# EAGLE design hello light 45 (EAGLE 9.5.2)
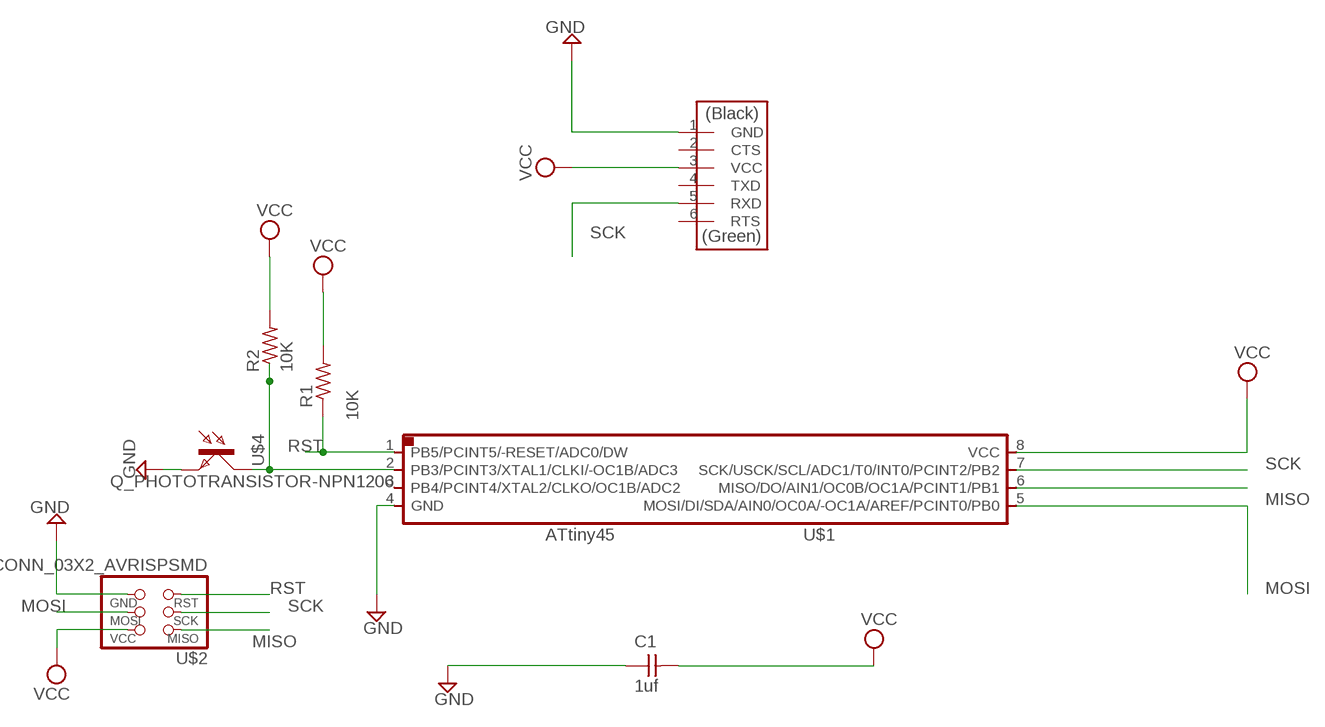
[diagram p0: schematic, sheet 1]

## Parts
C1  1uf  CAP_UNPOLARIZED  [C1206]
R1  10K  R1206FAB  [R1206FAB]
R2  10K  R1206FAB  [R1206FAB]
U$1  UC_ATTINY45SI  [SOIC8]
U$2  CONN_03X2_AVRISPSMD  [2X03SMD]
U$3  CONN_06_FTDI-SMD-HEADER  [1X06SMD]
U$4  Q_PHOTOTRANSISTOR-NPN1206  [OP1206]

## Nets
GND: C1.1 U$1.4(GND) U$2.6(GND) U$3.1(GND) U$4.EMITTER(E)
MISO: U$1.6(MISO/DO/AIN1/OC0B/OC1A/PCINT1/PB1) U$2.1(MISO)
MOSI: U$1.5(MOSI/DI/SDA/AIN0/OC0A/-OC1A/AREF/PCINT0/PB0) U$2.4(MOSI)
N$2: R2.1 U$1.2(PB3/PCINT3/XTAL1/CLKI/-OC1B/ADC3) U$4.COLLECTOR(C)
RST: R1.1 U$1.1(PB5/PCINT5/-RESET/ADC0/DW) U$2.5(RST)
SCK: U$1.7(SCK/USCK/SCL/ADC1/T0/INT0/PCINT2/PB2) U$2.3(SCK) U$3.5(RXD)
VCC: C1.2 R1.2 R2.2 U$1.8(VCC) U$2.2(VCC) U$3.3(VCC)
Unconnected: U$1.3(PB4/PCINT4/XTAL2/CLKO/OC1B/ADC2) U$3.2(CTS) U$3.4(TXD) U$3.6(RTS)

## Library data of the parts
C1 = fab:CAP_UNPOLARIZED
R1 R2 = fab:R: Resistor (US Symbol)
U$1 = fab:UC_ATTINY45
U$2 = fab:CONN_03X2_AVRISP
U$3 = fab:CONN_06_FTDI-SMD-HEADER
U$4 = fab:Q_PHOTOTRANSISTOR-NPN

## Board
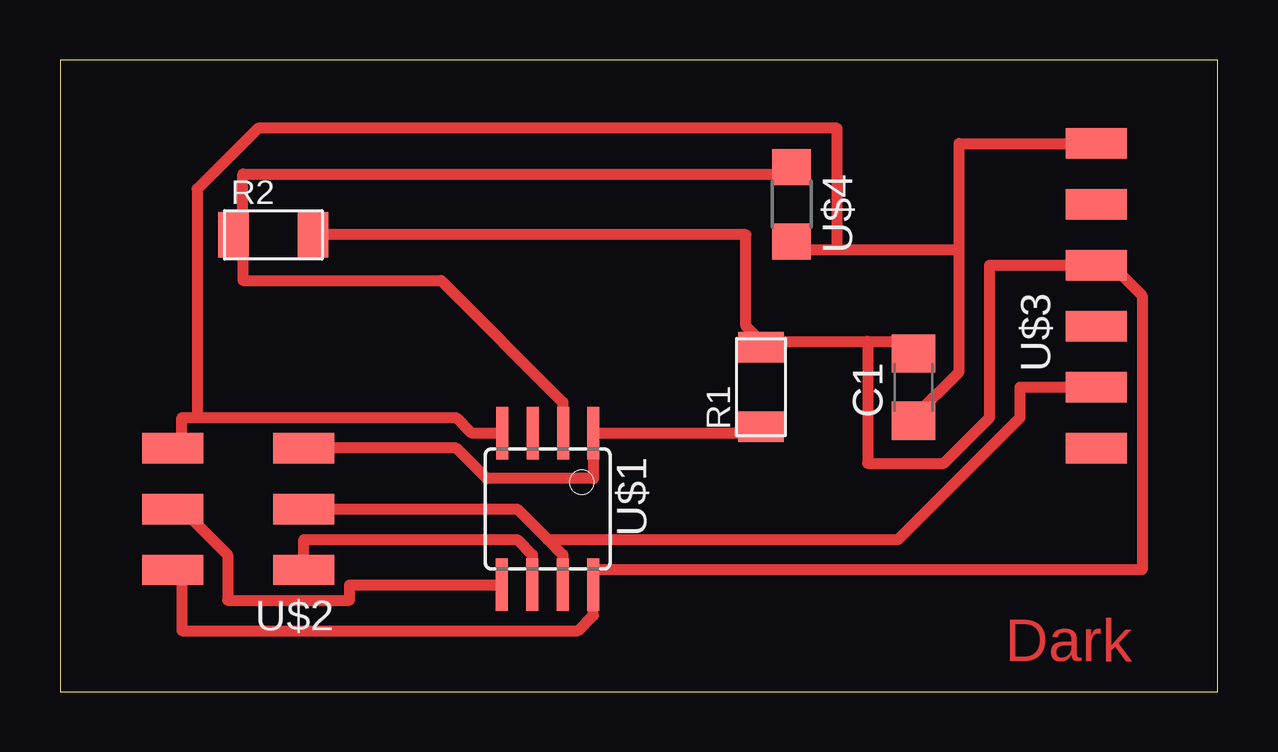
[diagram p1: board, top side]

Size 48.24 x 26.34 mm. Coordinates in mm from the lower left corner, seen from the top.
Outline: 0,0 48.24,0 48.24,26.34 0,26.34 0,0
Copper layers (1*16): Top 0.035mm / dielectric 1.5mm / Bottom 0.035mm
Design rules "fab-1": minimum track width 0.45mm, minimum drill 32mil, track to track 16mil, track to pad 16mil, pad to pad 16mil, via to via 16mil, smd to smd 6mil, copper to edge 16mil, drill to drill 16mil, minimum pad ring 10mil, minimum via ring 8mil, stop-mask expansion 4mil, vias tented up to drill 0mil, thermal gap 16mil

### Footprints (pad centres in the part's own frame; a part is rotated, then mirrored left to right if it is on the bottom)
C1206 = smd 1.6 x 1.8: 1 -1.4,0; 2 1.4,0
R1206FAB = smd 1.27 x 1.905: 1 -1.651,0; 2 1.651,0
SOIC8 = smd 0.5 x 2.2: 1 -1.905,-3.154; 2 -0.645,-3.154; 3 0.625,-3.154; 4 1.895,-3.154; 5 1.905,3.154; 6 0.635,3.154; 7 -0.635,3.154; 8 -1.905,3.154
2X03SMD = smd 2.54 x 1.27: 1 -2.54,2.54; 2 2.92,2.54; 3 -2.54,0; 4 2.92,0; 5 -2.54,-2.54; 6 2.92,-2.54
1X06SMD = smd 2.54 x 1.27: 1 0,6.35; 2 0,3.81; 3 0,1.27; 4 0,-1.27; 5 0,-3.81; 6 0,-6.35
OP1206 = smd 1.5 x 1.6: COLLECTOR -1.55,0; EMITTER 1.55,0

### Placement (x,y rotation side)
C1  35.56,12.7 90 top
R1  29.21,12.7 90 top
R2  8.89,19.05 0 top
U$1  20.32,7.62 180 top
U$2  7.62,7.62 180 top
U$3  43.18,16.51 0 top
U$4  30.48,20.32 270 top

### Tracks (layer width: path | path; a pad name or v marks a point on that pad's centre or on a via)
GND
  Top 0.45: 5.71,11.43 5.08,11.43 5.08,10.16 U$2.6 | 5.71,11.43 16.51,11.43 17.14,10.79 18.41,10.79 U$1.4 | 37.47,18.41 32.38,18.41 | 32.38,18.41 30.48,18.41 U$4.EMITTER | 37.47,18.41 37.47,13.34 35.56,11.43 C1.1 | U$3.1 37.47,22.86 37.47,18.41 | 5.71,11.43 5.71,20.95 8.25,23.49 32.38,23.49 32.38,18.41
MISO
  Top 0.45: U$1.6 19.68,5.71 19.05,6.35 10.16,6.35 U$2.1
MOSI
  Top 0.45: U$1.5 18.41,4.45 12.06,4.45 12.06,3.81 6.98,3.81 6.98,5.71 5.08,7.62 U$2.4
N$2
  Top 0.45: 7.62,19.05 7.62,21.59 30.48,21.59 U$4.COLLECTOR | 7.62,19.05 7.62,17.14 15.88,17.14 20.95,12.07 20.95,10.79 U$1.2 | 7.62,19.05 R2.1
RST
  Top 0.45: R1.1 29.21,10.79 22.23,10.79 U$1.1 22.23,8.89 17.78,8.89 16.51,10.16 U$2.5
SCK
  Top 0.45: U$1.7 20.95,5.71 20.32,6.35 | 20.32,6.35 19.05,7.62 U$2.3 | U$3.5 40,12.7 40,11.43 34.92,6.35 20.32,6.35
VCC
  Top 0.45: U$2.2 5.08,5.08 5.08,2.54 21.59,2.54 22.23,3.17 U$1.8 22.23,5.08 45.09,5.08 45.09,16.51 43.81,17.78 U$3.3 38.73,17.78 38.73,11.43 36.83,9.53 33.66,9.53 33.66,14.61 | 29.21,14.61 33.66,14.61 | 33.66,14.61 35.56,14.61 C1.2 | R2.2 28.57,19.05 28.57,15.24 29.21,14.61 | 29.21,14.61 R1.2

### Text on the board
Top: Dark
